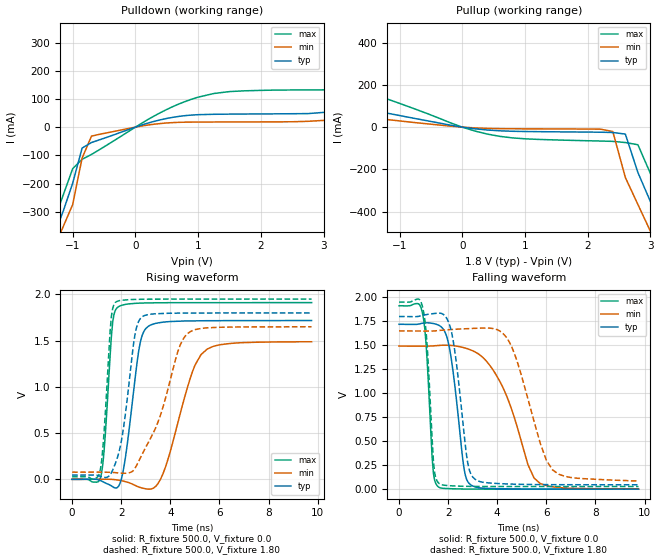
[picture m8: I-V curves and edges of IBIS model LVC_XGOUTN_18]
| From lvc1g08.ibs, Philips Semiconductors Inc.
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|   Model LVC_XGOUTN_18
[Model]   LVC_XGOUTN_18
Model_type   Output
Polarity   Non-Inverting
Vmeas =  0.9V
Cref  =  30.0pF
Rref  =  1.0k
Vref  =  0.0V
C_comp   3.40pF   2.23pF   4.36pF
[Model Spec]
| Note: The input and output voltage ratings may be exceeded if the input and
|   output current ratings are observed (please refer to the data sheet)
|   Subparameter   typ   min   max
| Timing Thresholds
Vmeas   0.9   0.825   0.975
|Ambient temperature:   25   85   -40
[Temperature Range]   25   85   -40
[Voltage Range]   1.80V   1.65V   1.95V
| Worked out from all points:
|   slope of the pulldown table from 0 to 0.27 V, typ, clamps not added: 14.4 ohm
|   slope of the pullup table from 0 to 0.27 V, typ, clamps not added: 27.3 ohm
|   rising waveform, R_fixture 500.0, V_fixture 0.0: 20-80 % time 476ps typ, 945ps min, 273ps max; typ from 0 V to 1.72 V
|   rising waveform, R_fixture 500.0, V_fixture 1.80: 20-80 % time 502ps typ, 1.16ns min, 266ps max; typ from 0.046 V to 1.8 V
|   falling waveform, R_fixture 500.0, V_fixture 0.0: 20-80 % time 464ps typ, 1.25ns min, 240ps max; typ from 1.72 V to 0 V
|   falling waveform, R_fixture 500.0, V_fixture 1.80: 20-80 % time 463ps typ, 1.06ns min, 249ps max; typ from 1.8 V to 0.046 V
|Process Range   nominal   slow   fast
[Pulldown]
| voltage   I(typ)   I(min)   I(max)
-5.5V     -4.525A    -4.561A    -4.482A
-1.45V    -520.9mA   -565.8mA   -470mA
-1.3V     -384.5mA   -430mA     -334mA
-1.15V    -297.4mA   -352.1mA   -240mA
-1V       -198.6mA   -274.3mA   -147.3mA
-850mV    -74.25mA   -109.7mA   -114.1mA
-700mV    -54.53mA   -31.75mA   -96.74mA
900mV     42.9mA     17.87mA    99.35mA
3.25V     59.57mA    28.49mA    143.3mA
5.5V      165.3mA    83.79mA    348.4mA
8.75V     350.2mA    185.6mA    696.7mA
11V       486.8mA    191.3mA    947.4mA
[Pullup]
| voltage   I(typ)   I(min)   I(max)
-9.35V    506.2mA    337.2mA    835.8mA
-8.55V    468.2mA    308.4mA    782.6mA
-4.75V    268.3mA    164.9mA    479.3mA
-2.75V    153.9mA    89.04mA    297.6mA
200mV     -7.848mA   -3.636mA   -18.36mA
2.4V      -25.33mA   -20.67mA   -67.34mA
2.6V      -32.86mA   -238.1mA   -72.8mA
2.8V      -214.4mA   -365.8mA   -83.27mA
3V        -352.1mA   -492.7mA   -219.4mA
3.2V      -516.1mA   -684.8mA   -373.7mA
3.4V      -715.5mA   -882.4mA   -569mA
7.45V     -4.682A    -4.863A    -4.503A
[Ramp]
| variable   typ   min   max
dV/dt_r   1.031V/476.124ps   892.838mV/945.379ps   1.147V/272.750ps
dV/dt_f   1.052V/463.597ps   938.224mV/1.060ns   1.154V/248.814ps
R_load = 500.0
[Rising Waveform]
R_fixture   = 500.0
V_fixture   = 0.0
V_fixture_min = 0.0
V_fixture_max = 0.0
| time   V(typ)   V(min)   V(max)
0s        9.233pV    355.8pV    3.068pV
1.15ns    -13.18mV   1.076mV    13.67mV
1.65ns    -79.96mV   -1.185mV   1.696V
1.85ns    -87.13mV   -7.511mV   1.86V
2.15ns    200.7mV    -23.74mV   1.891V
2.75ns    1.448V     -86.32mV   1.906V
3.1ns     1.655V     -106.5mV   1.908V
3.7ns     1.7V       60.79mV    1.91V
5.25ns    1.715V     1.35V      1.911V
9.75ns    1.718V     1.488V     1.912V
[Rising Waveform]
R_fixture   = 500.0
V_fixture   = 1.80
V_fixture_min = 1.65
V_fixture_max = 1.95
| time   V(typ)   V(min)   V(max)
0s        45.81mV    77.33mV    27.35mV
1.15ns    33.29mV    77.54mV    105.8mV
1.3ns     21mV       77.28mV    506.5mV
1.6ns     71.51mV    75.2mV     1.765V
1.8ns     200.6mV    70.91mV    1.921V
2.1ns     570mV      65.32mV    1.939V
2.55ns    1.551V     115.6mV    1.946V
2.85ns    1.758V     269.6mV    1.948V
4.7ns     1.799V     1.576V     1.95V
9.75ns    1.8V       1.65V      1.95V
[Falling Waveform]
R_fixture   = 500.0
V_fixture   = 0.0
V_fixture_min = 0.0
V_fixture_max = 0.0
| time   V(typ)   V(min)   V(max)
0s        1.719V     1.492V     1.912V
950ps     1.73V      1.491V     1.843V
1.4ns     1.727V     1.494V     168mV
1.6ns     1.711V     1.498V     24.25mV
2.05ns    1.477V     1.5V       5.372mV
2.65ns    211.1mV    1.474V     1.678mV
2.9ns     49.45mV    1.453V     1.036mV
4.1ns     4.367mV    1.126V     80.92uV
5.75ns    654.8uV    58.93mV    -12.22uV
9.75ns    -17.64uV   1.526mV    -2.035uV
[Falling Waveform]
R_fixture   = 500.0
V_fixture   = 1.80
V_fixture_min = 1.65
V_fixture_max = 1.95
| time   V(typ)   V(min)   V(max)
0s        1.8V       1.65V      1.95V
950ps     1.811V     1.649V     1.909V
1.4ns     1.83V      1.649V     301.6mV
1.65ns    1.835V     1.655V     56mV
2.15ns    1.625V     1.665V     34.75mV
2.8ns     271.2mV    1.673V     29.47mV
3.1ns     102.4mV    1.677V     28.56mV
4.5ns     53.4mV     1.53V      27.43mV
6.25ns    46.88mV    201.3mV    27.35mV
9.75ns    45.83mV    86.29mV    27.35mV
